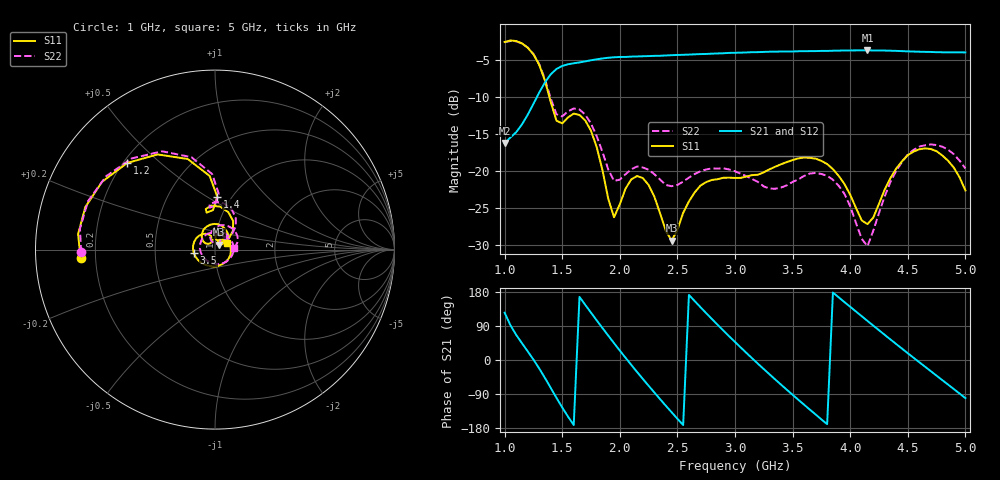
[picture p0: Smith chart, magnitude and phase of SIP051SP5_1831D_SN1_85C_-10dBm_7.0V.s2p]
# GHz  S  dB  R  50
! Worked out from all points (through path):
!   81 points, 1 GHz to 5 GHz, reference 50 ohm
!   highest |S21| = -3.63 dB at 4.15 GHz (marker M1); lowest = -16.2 dB at 1 GHz (marker M2)
!   lowest |S11| = -29.4 dB at 2.45 GHz (marker M3), VSWR 1.07, Z = 51.9 + j2.89 ohm
!   |S11| at or under -10 dB: 1.39 GHz to end of sweep
!   |S22| runs from -30.1 to -2.4 dB; largest |S21 - S12| = 0.002
!   S11 on the Smith chart (normalised r, x): 1 GHz: 0.14, -0.03; 1.2 GHz: 0.22, +0.39; 1.4 GHz: 0.86, +0.56; 3.5 GHz: 0.79, -0.03; 5 GHz: 1.13, +0.09
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1  -2.50 -176.6  -16.17 124.9  -16.15 125.0  -2.55 -178.9
1.2  -3.26 135.4  -12.36 23.1  -12.37 23.2  -3.25 132.4
1.4  -10.59 87.5  -6.88 -73.4  -6.87 -73.4  -10.11 86.2
1.55  -12.71 102.8  -5.52 -149.1  -5.51 -149.1  -11.87 96.8
1.7  -13.10 70.3  -5.12 145.5  -5.12 145.5  -12.31 67.3
1.85  -19.84 39.3  -4.73 84.2  -4.72 84.2  -17.39 43.4
1.95  -26.18 67.7  -4.57 44.4  -4.57 44.4  -21.27 55.5
2.05  -22.31 88.6  -4.52 5.8  -4.50 5.8  -20.37 68.4
2.2  -20.90 59.3  -4.43 -49.9  -4.43 -49.9  -19.46 54.9
2.35  -25.68 36.4  -4.36 -103.4  -4.34 -103.3  -21.10 44.2
2.45  -29.35 54.7  -4.29 -138.0  -4.29 -138.0  -21.99 45.9
2.6  -24.05 64.1  -4.21 171.7  -4.19 171.8  -20.83 44.7
2.75  -21.43 27.5  -4.12 123.6  -4.11 123.6  -19.72 27.2
3  -20.88 -48.1  -3.96 47.6  -3.94 47.5  -19.97 -19.0
3.25  -20.11 -117.0  -3.84 -24.0  -3.84 -24.1  -22.02 -90.7
3.5  -18.46 -170.9  -3.79 -91.8  -3.78 -91.9  -21.41 174.3
3.7  -18.27 148.6  -3.73 -143.8  -3.72 -143.9  -20.20 115.0
3.9  -20.59 114.1  -3.67 165.5  -3.66 165.4  -21.93 71.1
4.15  -27.11 126.4  -3.63 103.1  -3.62 103.2  -30.09 85.0
4.35  -20.88 141.6  -3.68 54.0  -3.69 54.1  -21.40 108.5
4.65  -16.88 91.5  -3.84 -17.8  -3.85 -17.8  -16.46 58.6
5  -22.56 30.5  -3.91 -100.6  -3.91 -100.7  -19.59 4.6
